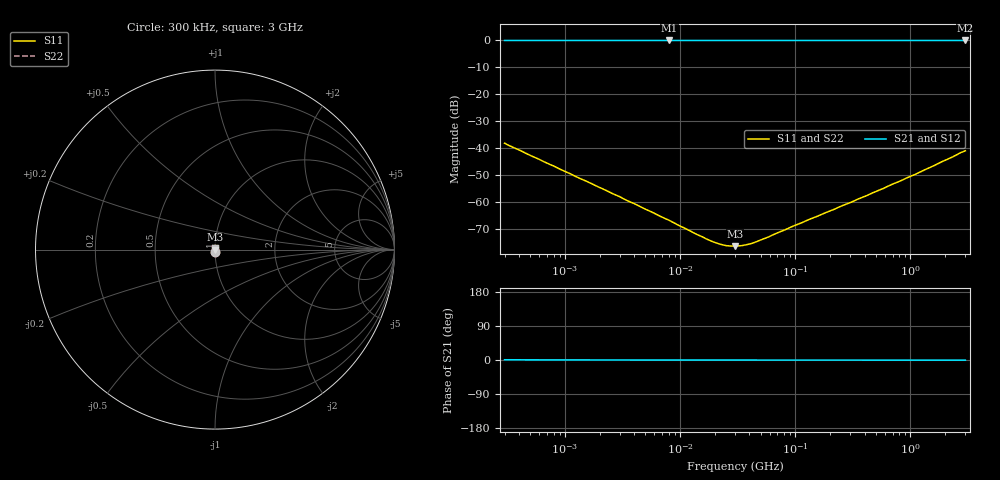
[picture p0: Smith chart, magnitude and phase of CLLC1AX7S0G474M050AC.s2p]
! S-Parameter Data Generated by TDK Corporation
! Copyright(C) 2022 TDK Corporation.
! All Rights Reserved.
! TDK P/N: CLLC1AX7S0G474M050AC (Multilayer Ceramic Chip Capacitor)
! Property: C=470nF
! Size(LxWxT): 1.6x0.8x0.5mm
! Model Type: s2p (Touchstone File Format Version 1.0)
! Frequency: DC=Yes Start=0.3MHz Stop=3000MHz 402points Log-sweep
! Model Generated on Apr. 15, 2022
! Port Assignments:
!  1 ---| |--- 2
! Applicable Conditions:
!  Temperature = 25 degC
!  DC Bias Voltage = 0 V
!  Small Signal Operation
! Terms and conditions regarding TDK Simulation Models
! (1)This simulation model is being provided solely for informational purposes. Please refer to the specifications of the products in terms of detailed characteristics of such products.
! (2)In no event shall TDK Corporation of any of its subsidiaries be liable for any loss or damage arising, directly or indirectly,
!  From any information contained in this simulation model, including, but not limited to loss or damages arising from any inaccuracies, omissions or errors in connection with such information.
! (3)Any and all copyrights on this simulation model are owned by TDK Corporation.
!  Duplication or redistribution of this simulation model without prior written permission from TDK Corporation is prohibited.
! (4)This simulation model is subject to any modification or change without any prior notice.
! (5)Neither TDK Corporation nor any of its subsidiaries shall make any warranty, express or implied,
!  Including but not limited to the correctness, implied warranties of merchantability and fitness for a particular purpose with respect to this simulation models.
! (6)The use of this simulation model shall be deemed to have consented to the terms and conditions hereof.
# Hz S MA R 50
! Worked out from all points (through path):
!   401 points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, 300 kHz to 3 GHz, reference 50 ohm
!   highest |S21| = 0.00 dB at 8.075 MHz (marker M1); lowest = 0.0 dB at 3 GHz (marker M2)
!   lowest |S11| = -76.4 dB at 30 MHz (marker M3), VSWR 1.00, Z = 50 - j0.000739 ohm
!   |S11| at or under -10 dB: start of sweep to end of sweep
!   |S22| runs from -76.4 to -38.1 dB; largest |S21 - S12| = 0
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300000  0.01238 -88.0  0.9996 0.7  0.9996 0.7  0.01238 -88.0
404689  0.009201 -88.0  0.9997 0.5  0.9997 0.5  0.009201 -88.0
1403210  0.002647 -86.3  0.9998 0.2  0.9998 0.2  0.002647 -86.3
4141150  0.0009066 -80.9  0.9999 0.1  0.9999 0.1  0.0009066 -80.9
6563280  0.00056 -75.5  0.9999 0.0  0.9999 0.0  0.00056 -75.5
8074600  0.000456 -72.3  0.9999 0.0  0.9999 0.0  0.000456 -72.3
1.37126e7  0.0002564 -56.7  0.9999 0.0  0.9999 0.0  0.0002564 -56.7
1.93696e7  0.0001827 -37.9  0.9999 0.0  0.9999 0.0  0.0001827 -37.9
2.43849e7  0.0001574 -19.6  0.9999 0.0  0.9999 0.0  0.0001574 -19.6
2.67375e7  0.0001534 -11.9  0.9998 0.0  0.9998 0.0  0.0001534 -11.9
3e7  0.0001517 -2.8  0.9998 0.0  0.9998 0.0  0.0001517 -2.8
3.60679e7  0.0001583 13.6  0.9998 -0.0  0.9998 -0.0  0.0001583 13.6
4.33632e7  0.0001749 26.7  0.9998 -0.0  0.9998 -0.0  0.0001749 26.7
5.71638e7  0.00022 42.0  0.9998 -0.0  0.9998 -0.0  0.00022 42.0
9.48683e7  0.0003544 58.7  0.9998 -0.0  0.9998 -0.0  0.0003544 58.7
1.40321e8  0.000501 65.8  0.9998 -0.0  0.9998 -0.0  0.000501 65.8
3e8  0.0009752 74.5  0.9997 -0.1  0.9997 -0.1  0.0009752 74.5
6.56328e8  0.002025 79.7  0.9996 -0.1  0.9996 -0.1  0.002025 79.7
1.14057e9  0.003379 81.7  0.9995 -0.2  0.9995 -0.2  0.003379 81.7
2.27573e9  0.006742 82.0  0.9991 -0.4  0.9991 -0.4  0.006742 82.0
2.67375e9  0.00807 82.1  0.9989 -0.5  0.9989 -0.5  0.00807 82.1
3e9  0.008977 81.9  0.9988 -0.5  0.9988 -0.5  0.008977 81.9
